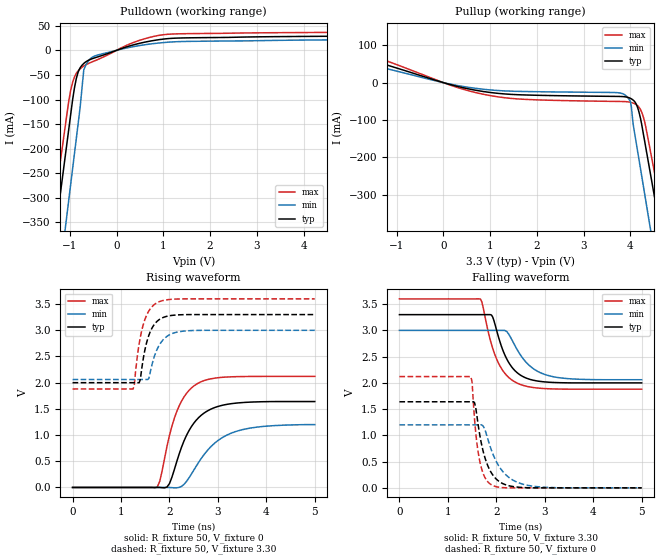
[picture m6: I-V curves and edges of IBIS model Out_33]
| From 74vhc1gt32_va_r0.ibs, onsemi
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|//////////////////////////////////////////////////////////////////////////////
|//////////////////////////////////////////////////////////////////////////////
[Model] Out_33
Model_type Output
Polarity Non-Inverting
Vmeas = 1.65
Vref = 3.30
Rref = 1k
Cref = 15pF
|  variable   typ   min   max
C_comp   3.9pF   3.9pF   3.9pF
|//////////////////////////////////////////////////////////////////////////////
[Temperature Range]   25   125   -55
|//////////////////////////////////////////////////////////////////////////////
[Voltage Range]   3.30V   3.00V   3.60V
|//////////////////////////////////////////////////////////////////////////////
[Pulldown Reference]   0V   0V   0V
|//////////////////////////////////////////////////////////////////////////////
[Pullup Reference]   3.30V   3.00V   3.60V
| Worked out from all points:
|   slope of the pulldown table from 0 to 0.495 V, typ, clamps not added: 34.5 ohm
|   slope of the pullup table from 0 to 0.495 V, typ, clamps not added: 31.8 ohm
|   falling waveform, R_fixture 50, V_fixture 3.30: 20-80 % time 362ps typ, 475ps min, 374ps max; typ from 3.3 V to 2 V
|   falling waveform, R_fixture 50, V_fixture 0: 20-80 % time 264ps typ, 391ps min, 158ps max; typ from 1.64 V to 0 V
|   rising waveform, R_fixture 50, V_fixture 0: 20-80 % time 484ps typ, 664ps min, 409ps max; typ from 0 V to 1.64 V
|   rising waveform, R_fixture 50, V_fixture 3.30: 20-80 % time 212ps typ, 248ps min, 212ps max; typ from 2 V to 3.3 V
|//////////////////////////////////////////////////////////////////////////////
[Pulldown]
|   Voltage   I(typ)   I(min)   I(max)
-3.3V     -1.847A    -2.055A    -1.688A
-1.4V     -435.6mA   -596.3mA   -361.6mA
-1.28V    -348.3mA   -503.6mA   -279.2mA
-1.14V    -246.4mA   -395.4mA   -183.3mA
-1.06V    -188.1mA   -333.6mA   -128.5mA
-980mV    -129.8mA   -271.7mA   -80.83mA
-860mV    -56.93mA   -178.9mA   -46.63mA
-700mV    -26.48mA   -39.38mA   -31.73mA
-460mV    -15.06mA   -11.28mA   -21mA
400mV     12.12mA    8.241mA    17.34mA
1.1V      23.86mA    16.57mA    32.69mA
6.6V      32.18mA    24.05mA    41.22mA
|//////////////////////////////////////////////////////////////////////////////
[Pullup]
|   Voltage   I(typ)   I(min)   I(max)
-3.3V     120mA      97.93mA    143.8mA
840mV     -23.43mA   -17.44mA   -30.74mA
3.84V     -37.34mA   -29.79mA   -50.5mA
4V        -41.93mA   -50.86mA   -52.46mA
4.06V     -46.73mA   -111.8mA   -54.68mA
4.16V     -68.45mA   -187.5mA   -62.18mA
4.28V     -138.5mA   -278.2mA   -92.76mA
4.42V     -237.4mA   -384.1mA   -177.5mA
4.58V     -350.4mA   -505.2mA   -282.4mA
4.66V     -406.9mA   -565.7mA   -334.9mA
4.78V     -491.6mA   -656.4mA   -413.6mA
6.6V      -1.782A    -2.037A    -1.613A
|//////////////////////////////////////////////////////////////////////////////
|//////////////////////////////////////////////////////////////////////////////
[Ramp]
|  variable   typ   min   max
dV/dt_f   7.800E-01/3.750E-10  5.640E-01/4.750E-10  1.032E+00/3.750E-10
dV/dt_r   9.840E-01/5.000E-10  7.200E-01/7.000E-10  1.272E+00/4.000E-10
R_load = 50
|/////////////////////////////////////////////////////////////////////////////
[Falling Waveform]
R_fixture = 50
V_fixture = 3.30
V_fixture_min = 3.00
V_fixture_max = 3.60
C_fixture = 0p
|   time   V(typ)   V(min)   V(max)
0s        3.3V       3V         3.6V
1.675ns   3.3V       3V         3.595V
1.725ns   3.3V       3V         3.452V
1.9ns     3.293V     3V         2.735V
2.025ns   2.939V     3.001V     2.415V
2.225ns   2.439V     2.968V     2.131V
2.5ns     2.147V     2.53V      1.969V
2.8ns     2.044V     2.249V     1.907V
3.2ns     2.007V     2.113V     1.884V
5ns       2V         2.06V      1.88V
|//////////////////////////////////////////////////////////////////////////////
[Falling Waveform]
R_fixture = 50
V_fixture = 0
C_fixture = 0p
|   time   V(typ)   V(min)   V(max)
0s        1.64V      1.2V       2.12V
1.475ns   1.64V      1.2V       2.121V
1.5ns     1.64V      1.2V       2.011V
1.55ns    1.625V     1.2V       1.31V
1.65ns    1.053V     1.2V       544mV
1.775ns   545.7mV    1.081V     179.3mV
1.925ns   247.5mV    653.9mV    45.05mV
2.2ns     56.43mV    245.4mV    1.175mV
2.6ns     4.113mV    57.78mV    0V
5ns       0V         0V         0V
|//////////////////////////////////////////////////////////////////////////////
[Rising Waveform]
R_fixture = 50
V_fixture = 0
C_fixture = 0p
|   time   V(typ)   V(min)   V(max)
0s        0V         0V         0V
1.75ns    949.4uV    47.02uV    10.52mV
1.8ns     366.4uV    48.36uV    118.2mV
1.95ns    8.635mV    808.8uV    788mV
2.15ns    490.5mV    -6.431mV   1.446V
2.4ns     1.079V     178.1mV    1.849V
2.65ns    1.373V     544.7mV    2.017V
3ns       1.546V     894.9mV    2.094V
3.4ns     1.613V     1.077V     2.115V
5ns       1.64V      1.2V       2.12V
|//////////////////////////////////////////////////////////////////////////////
[Rising Waveform]
R_fixture = 50
V_fixture = 3.30
V_fixture_min = 3.00
V_fixture_max = 3.60
C_fixture = 0p
|   time   V(typ)   V(min)   V(max)
0s        2V         2.06V      1.88V
1.25ns    2V         2.06V      1.88V
1.275ns   2V         2.06V      1.961V
1.375ns   1.999V     2.06V      2.745V
1.475ns   2.54V      2.06V      3.155V
1.575ns   2.904V     2.082V     3.37V
1.675ns   3.095V     2.462V     3.482V
1.8ns     3.211V     2.733V     3.549V
2.325ns   3.299V     2.987V     3.6V
5ns       3.3V       3V         3.6V
